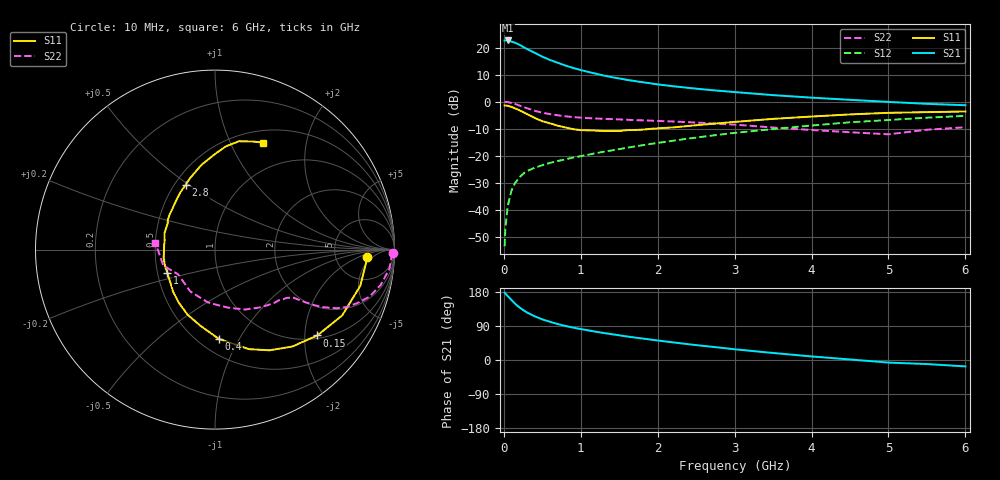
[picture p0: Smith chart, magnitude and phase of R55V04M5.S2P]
! SIEMENS Small Signal Semiconductors
! BFR183
! Si NPN RF Bipolar Junction Transistor in SOT23
! VCE = 5 V  IC = 4.5 mA
! Common Emitter S-Parameters:  May  1996
# GHz  S  MA  R  50
!  f  S11  S21  S12  S22
! GHz  MAG  ANG  MAG  ANG  MAG  ANG  MAG  ANG
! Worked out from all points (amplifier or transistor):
!   36 points, 10 MHz to 6 GHz, reference 50 ohm
!   highest |S21| = 22.6 dB at 50 MHz (marker M1)
!   |S21| within 3 dB of that: start of sweep to 291.8 MHz
!   unconditionally stable (mu >= 1): 1.098 GHz to 2.689 GHz
!   at 250 MHz: K = 0.39, MSG = 23.5 dB, |S12| = -26.8 dB
!   at 1.4 GHz: K = 1.06, MAG = 12.1 dB, |S12| = -18.1 dB
!   at 6 GHz: K = 0.88, MSG = 2.0 dB, |S12| = -5.3 dB
!   S11 on the Smith chart (normalised r, x): 10 MHz: 11, -3; 150 MHz: 1.08, -2.31; 400 MHz: 0.62, -0.83; 1 GHz: 0.56, -0.16; 2.8 GHz: 0.57, +0.49; 6 GHz: 0.64, +1.34
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0.01  0.8477 -2.9  13.47 177.9  0.0021 90.7  0.9904 -1.2
0.02  0.8439 -5.5  13.53 175.2  0.0044 83.5  0.9844 -2.5
0.05  0.8343 -14.0  13.53 168.7  0.0115 81.2  0.978 -6.3
0.1  0.7979 -27.4  12.89 158.3  0.0226 75.9  0.9434 -12.1
0.15  0.7441 -40.0  12.19 147.7  0.0317 70.0  0.8993 -17.0
0.2  0.691 -51.4  11.31 139.3  0.0391 65.8  0.8456 -20.7
0.25  0.6378 -61.6  10.29 132.0  0.0457 61.7  0.7966 -23.7
0.3  0.5863 -71.1  9.447 125.5  0.0516 59.7  0.7535 -25.7
0.4  0.4982 -87.5  8.024 115.5  0.0595 56.3  0.6761 -28.3
0.5  0.4328 -100.6  6.768 107.1  0.0663 55.1  0.6207 -29.5
0.6  0.3944 -112.6  5.896 100.8  0.0731 54.5  0.585 -30.2
0.7  0.3575 -124.6  5.226 94.9  0.0791 54.4  0.5576 -30.7
0.8  0.3317 -134.5  4.649 89.9  0.0854 54.8  0.5345 -31.1
1  0.2957 -153.6  3.832 81.6  0.0974 56.2  0.5038 -32.0
1.1  0.2934 -161.8  3.529 78.1  0.1039 56.9  0.4939 -32.9
1.6  0.2953 162.5  2.523 62.1  0.1392 57.8  0.4598 -37.7
2.2  0.3319 134.6  1.922 46.5  0.1884 56.9  0.4278 -46.3
2.8  0.3965 114.3  1.582 32.9  0.2435 53.2  0.3861 -58.2
3.5  0.478 99.1  1.315 18.5  0.3096 46.3  0.3304 -77.9
4.5  0.5778 84.1  1.077 1.4  0.4129 34.8  0.2705 -120.7
5.5  0.637 71.0  0.908 -10.7  0.503 22.3  0.3009 -162.8
6  0.6546 65.7  0.855 -16.9  0.5444 14.1  0.3343 173.7
